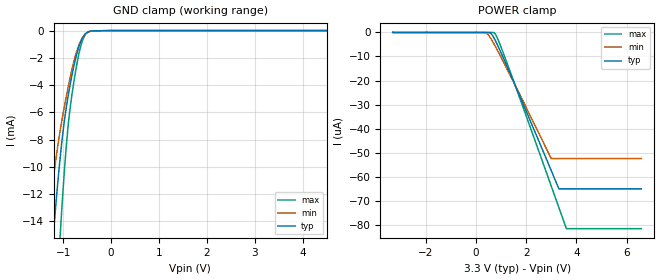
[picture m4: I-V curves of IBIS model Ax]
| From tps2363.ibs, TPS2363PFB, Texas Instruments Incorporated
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|   Ax MODEL
[Model]   Ax
Model_type   Input
|   Valid for A0,A1,A2
Vinl = 0.8V
Vinh = 2.0V
|   typ   min   max
C_comp   2.571pF   2.706pF   2.445pF
[Voltage Range]   3.300V   3.000V   3.600V
|Junction Temperature
[Temperature Range]   40.0   125.0   -40.0
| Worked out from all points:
|   GND clamp passes 1 mA (typ) near -0.65 V on its own axis
[GND Clamp]
|   Voltage   I(typ)   I(min)   I(max)
-3.3V     -183.6mA   -124.9mA   -260mA
-1.34V    -21.72mA   -15.04mA   -35.42mA
-1.201V   -14.92mA   -10.79mA   -24.43mA
-1.063V   -9.367mA   -7.36mA    -15.14mA
-1.053V   -9.026mA   -7.148mA   -14.55mA
-973.5mV  -6.614mA   -5.573mA   -10.3mA
-914.1mV  -5.196mA   -4.481mA   -7.686mA
-815.1mV  -3.265mA   -2.823mA   -4.682mA
-716.1mV  -1.724mA   -1.511mA   -2.515mA
-617.1mV  -677.5uA   -648uA     -947.5uA
-468.6mV  -77.81uA   -100.9uA   -85.49uA
6.58V     0A         0A         0A
[POWER Clamp]
|   Voltage   I(typ)   I(min)   I(max)
-3.3V     901.4pA    5.395nA    161.9pA
343.2mV   -24.75nA   -67.64nA   -23.57nA
452.1mV   -27.76nA   -558.2nA   -23.63nA
580.8mV   -270.3nA   -2.278uA   -23.83nA
650.1mV   -1.045uA   -3.467uA   -27.99nA
739.2mV   -2.644uA   -5.111uA   -263.4nA
867.9mV   -5.393uA   -7.607uA   -2.646uA
1.185V    -12.77uA   -14.03uA   -11.16uA
2.996V    -57.33uA   -52.4uA    -63.77uA
3.303V    -64.97uA   -52.4uA    -72.78uA
3.6V      -64.97uA   -52.4uA    -81.51uA
6.58V     -64.97uA   -52.4uA    -81.51uA
